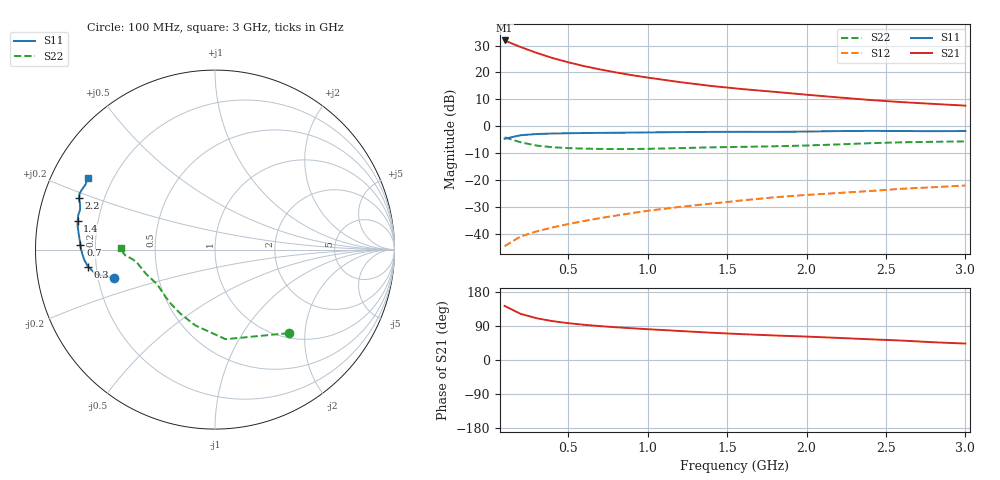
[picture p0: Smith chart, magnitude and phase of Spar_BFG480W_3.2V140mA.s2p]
! Filename: 3_2140BFG480.001
! Title: BFG480W
! Bias: Vce=3.2V; Ic=140mA
! Company: NXP Semiconductors NL
! User: Quality&Reliability T&D
! Measure time: 10 Nov 1999 / 11:58:47
#  MHz  S  MA  R 50
! Freq  S11  S21  S12  S22  :
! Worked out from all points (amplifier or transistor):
!   20 points, 100 MHz to 3 GHz, reference 50 ohm
!   highest |S21| = 31.9 dB at 100 MHz (marker M1)
!   |S21| within 3 dB of that: start of sweep to 226.4 MHz
!   unconditionally stable (mu >= 1): 439.2 MHz to end of sweep
!   at 400 MHz: K = 0.98, MSG = 31.5 dB, |S12| = -37.7 dB
!   at 1.2 GHz: K = 1.14, MAG = 21.0 dB, |S12| = -30.0 dB
!   at 3 GHz: K = 1.10, MAG = 12.9 dB, |S12| = -22.1 dB
!   S11 on the Smith chart (normalised r, x): 100 MHz: 0.27, -0.13; 300 MHz: 0.17, -0.06; 700 MHz: 0.14, +0.02; 1.4 GHz: 0.12, +0.10; 2.2 GHz: 0.11, +0.18; 3 GHz: 0.11, +0.26
100  0.5831 -164.2  39.28 142.6  0.005868 66.9  0.6203 -48.6
200  0.6784 -168.4  29.69 121.8  0.008895 60.4  0.5027 -83.2
300  0.7138 -172.4  23.15 110.3  0.01102 61.1  0.4366 -104.5
400  0.7305 -175.4  18.54 102.7  0.01306 63.5  0.4058 -118.2
500  0.7388 -177.9  15.44 97.2  0.01512 66.1  0.391 -127.7
600  0.7458 -180.0  13.1 92.9  0.01725 68.2  0.3827 -134.5
700  0.7503 178.2  11.38 89.4  0.01949 70.2  0.3778 -139.6
800  0.7544 176.4  10 86.4  0.02174 71.7  0.3755 -143.8
900  0.7598 174.7  8.894 83.8  0.02413 73.4  0.3759 -147.4
1000  0.7652 173.2  8.013 81.3  0.02667 74.1  0.3791 -150.6
1200  0.7759 170.5  6.617 76.6  0.03148 75.4  0.3908 -155.7
1400  0.7823 168.3  5.598 72.0  0.03628 76.0  0.4039 -159.5
1600  0.7855 165.9  4.885 68.1  0.04179 76.5  0.4128 -162.5
1800  0.7842 163.4  4.346 64.7  0.04768 76.7  0.4227 -165.8
2000  0.7939 161.4  3.847 61.8  0.05264 77.2  0.4369 -169.7
2200  0.8105 159.3  3.428 58.3  0.05724 77.0  0.4579 -172.9
2400  0.8166 157.5  3.068 54.6  0.06225 76.3  0.4825 -175.0
2600  0.8131 155.7  2.802 51.3  0.06851 75.4  0.5017 -176.4
2800  0.8075 153.4  2.595 46.8  0.07329 73.9  0.512 -178.1
3000  0.8126 150.7  2.41 43.4  0.0788 73.0  0.5211 179.1
